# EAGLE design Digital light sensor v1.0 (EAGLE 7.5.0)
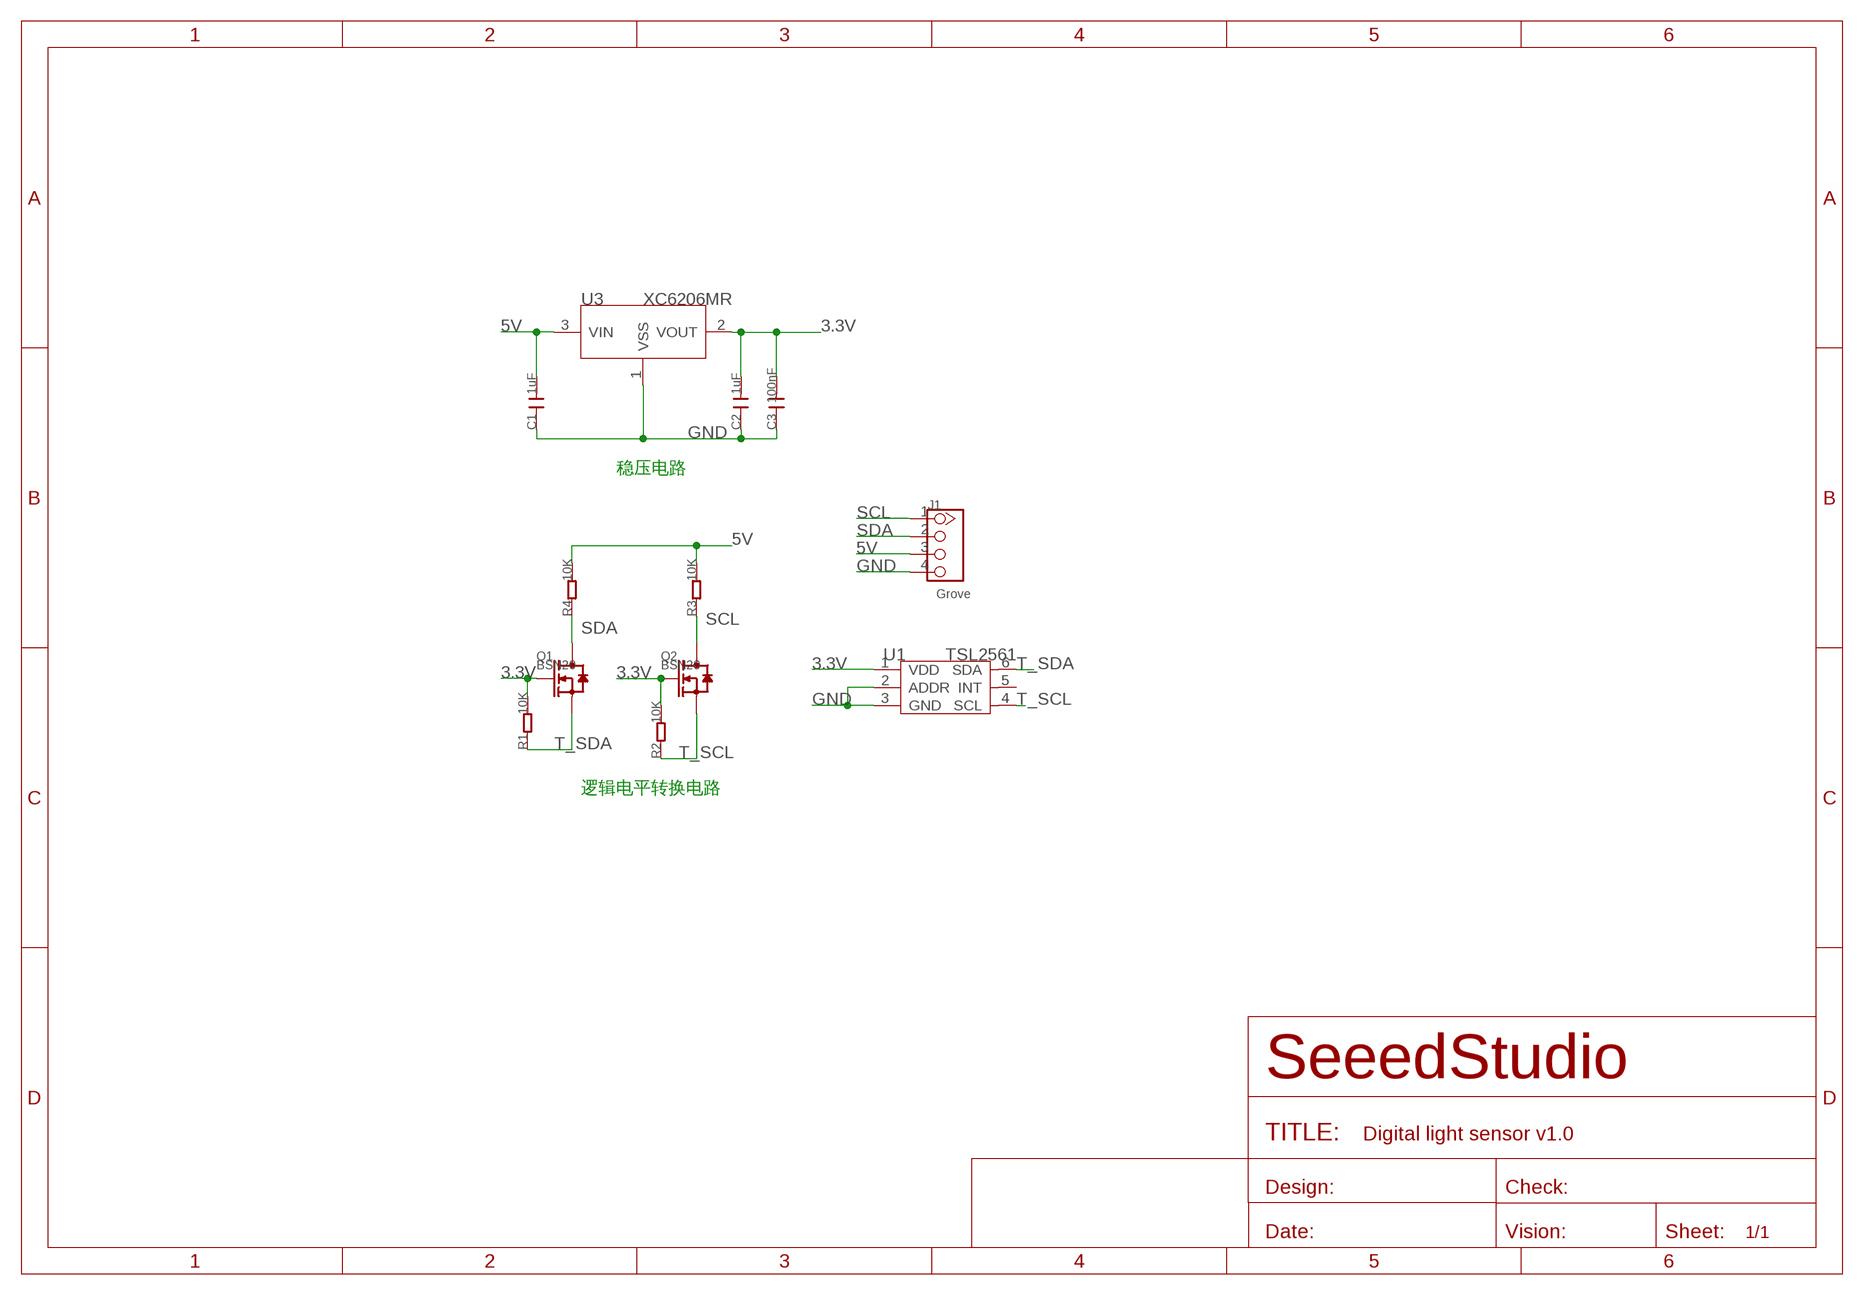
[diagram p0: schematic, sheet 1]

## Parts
C1  1uF  C-0603  [C0603]
C2  1uF  C-0603  [C0603]
C3  100nF  C-0603  [C0603]
J1  Grove  TWIG-4P-2.0-2.0  [4P-2.0]
Q1  BSN20  MOSFET-N'SOT23'  [SOT23]
Q2  BSN20  MOSFET-N'SOT23'  [SOT23]
R1  10K  R-0603  [R0603]
R2  10K  R-0603  [R0603]
R3  10K  R-0603  [R0603]
R4  10K  R-0603  [R0603]
U1  TSL2561  TSL2561T  [TMB-6]
U3  XC6206MR  [SOT23]

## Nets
3.3V: C2.2 C3.2 Q1.1(G) Q2.1(G) R1.2 R2.2 U1.1(VDD) U3.2(VOUT)
5V: C1.2 J1.3 R3.2 R4.2 U3.3(VIN)
GND: C1.1 C2.1 C3.1 J1.4 U1.2(ADDR) U1.3(GND) U3.1(VSS)
SCL: J1.1 Q2.3(D) R3.1
SDA: J1.2 Q1.3(D) R4.1
T_SCL: Q2.2(S) R2.1 U1.4(SCL)
T_SDA: Q1.2(S) R1.1 U1.6(SDA)
Unconnected: U1.5(INT)

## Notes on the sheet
- 稳压电路
- 逻辑电平转换电路

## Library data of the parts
C1-C3 = Discrete:C*: Ceramic Capacitors
J1 = Connector:TWIG-4P-2.0
Q1 Q2 = Discrete:MOSFET-N: IRLL014: http://www.vishay.com/docs/91319/sihll014.pdf
R1-R4 = Discrete:R*
U1 = template:TSL2561: Light-TO-Digital Converter
U3 = IC:XC6206: LOW ESR Cap.Compatible Positive Voltage Regulators

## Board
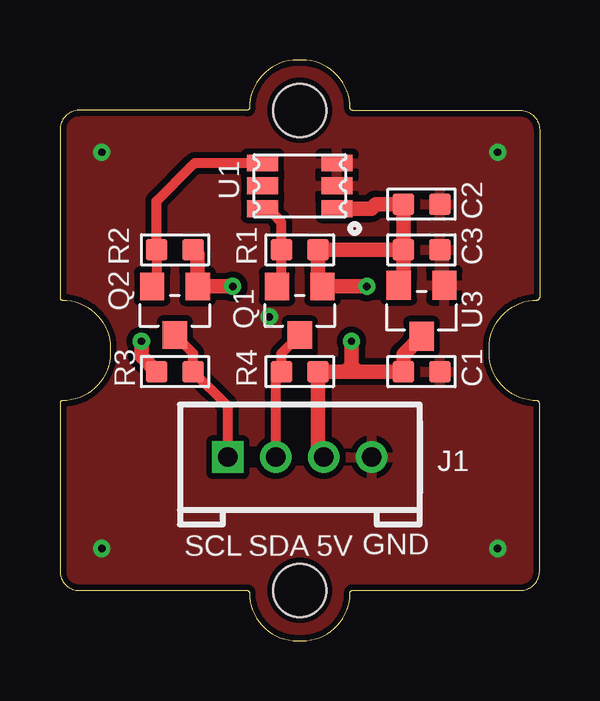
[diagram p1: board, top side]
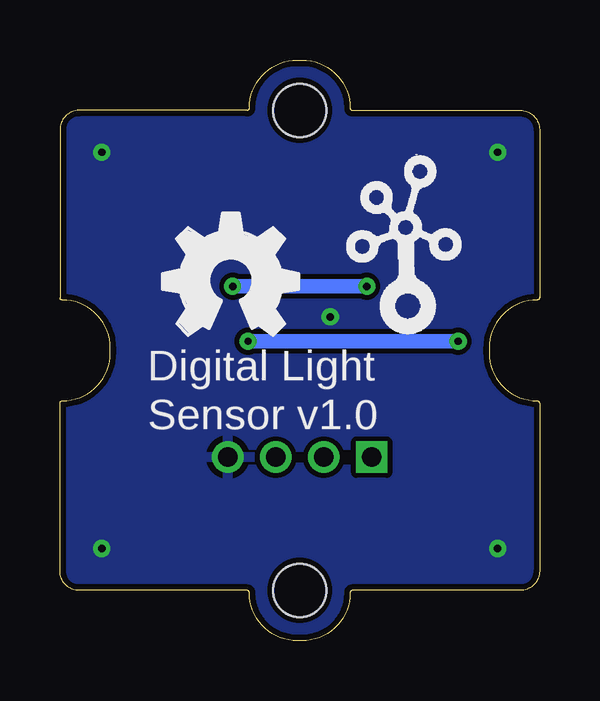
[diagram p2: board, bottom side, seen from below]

Size 20 x 24.2 mm. Coordinates in mm from the lower left corner, seen from the top.
Copper layers (1*16): Top 0.035mm / dielectric 1.5mm / Bottom 0.035mm
Design rules "default": minimum track width 10mil, minimum drill 12mil, track to track 8mil, track to pad 8mil, pad to pad 8mil, via to via 8mil, smd to smd 0mil, copper to edge 10mil, drill to drill 8mil, minimum pad ring 10mil, minimum via ring 8mil, stop-mask expansion 4mil, vias tented up to drill 25mil, thermal gap 10mil

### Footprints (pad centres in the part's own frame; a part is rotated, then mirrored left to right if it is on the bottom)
C0603 = smd 0.889 x 0.889: 1 -0.762,0; 2 0.762,0
4P-2.0 = drill 0.8 pad 1.27 square: 1 -3,0 | drill 0.8 pad 1.27: 2 -1,0; 3 1,0; 4 3,0
SOT23 = smd 1.016 x 1.143: 1 -0.95,-1.016; 2 0.95,-1.016; 3 0,1.016
R0603 = smd 0.889 x 0.889: 1 -0.762,0; 2 0.762,0
TMB-6 = smd 1.3 x 0.7: 1 -1.55,0.95; 2 -1.55,0; 3 -1.55,-0.95; 4 1.55,-0.95; 5 1.55,0; 6 1.55,0.95
SOT23' = smd 1.016 x 1.2: 1 -0.95,-1.06; 2 0.95,-1.06; 3 0,1.06
1U-DIM-W/-DRILL = hole 2.2: 0,-10; 0,10

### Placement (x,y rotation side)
C1  15.08,11.21 180 top
C2  15.08,18.2 180 top
C3  15.08,16.29 180 top
J1  10,7.65 0 top
Q1  10,13.75 180 top
Q2  4.79,13.75 180 top
R1  10,16.29 0 top
R2  4.79,16.29 0 top
R3  4.79,11.21 180 top
R4  10,11.21 0 top
U1  10,18.96 180 top
U3  XC6206MR  [SOT23']  15.08,13.75 180 top
U$2  [1U-DIM-W/-DRILL]  10,12.1 0 top
U$3  [TWIGLOGO]  5.55,13.75 0 bottom
U$4  [OSHW_FILLX200_NOTEXT]  15.71,12.73 0 bottom

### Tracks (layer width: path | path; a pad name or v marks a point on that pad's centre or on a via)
3.3V  (via drill 0.3 pad 0.64)
  Top 0.61: v7.21,14.77 Q2.1 5.74,16.1 R2.2 | v12.79,14.77 Q1.1 10.76,14.96 R1.2 C3.2 | C3.2 14.32,15 U3.2 | C3.2 C2.2 13.18,18.2 12.99,18.01 U1.1
  Bottom 0.61: v7.21,14.77 v12.79,14.77
5V  (via drill 0.3 pad 0.64)
  Top 0.61: U3.3 14.32,11.93 C1.2 12.41,11.21 | 12.41,11.21 12.16,11.21 | 12.16,11.21 11.9,11.21 | 11.9,11.21 R4.2 10.76,7.89 J1.3 | v12.16,12.48 12.16,11.72 | 12.16,11.72 12.16,11.21 | v3.4,12.48 3.4,11.85 R3.2 | 12.16,11.72 12.16,11.46 | 12.16,11.46 11.9,11.21 | 12.16,11.72 12.16,11.46 | 12.16,11.46 12.41,11.21
  Bottom 0.61: v3.4,12.48 v12.16,12.48 v3.4,12.48
GND  (via drill 0.3 pad 0.64)
  other vias: 1.74,20.36 18.26,20.36 18.26,3.84 1.74,3.84 8.73,13.5
  pour Bottom: -0.79,24.8 20.8,24.8 20.8,-0.6 -0.79,-0.6
  pour Top (isolate 0.254): -0.79,24.8 20.8,24.8 20.8,-0.6 -0.79,-0.6
SCL
  Top 0.406: Q2.3 5.55,11.97 R3.1 7,9.77 J1.1
SDA
  Top 0.406: R4.1 9.24,11.97 Q1.3 | 9,10.97 R4.1 | J1.2 9,10.97 | 9,10.97 R4.1
T_SCL
  Top 0.406: Q2.2 4.03,14.96 R2.1 4.03,18.32 5.55,19.85 5.62,19.91 U1.4
T_SDA
  Top 0.406: Q1.2 9.11,14.77 9.24,14.89 R1.1 9.24,17.43 9.11,17.56 8.66,18.01 U1.6

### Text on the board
tPlace: SCL | SDA | 5V | GND
bPlace: Digital Light | Sensor v1.0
